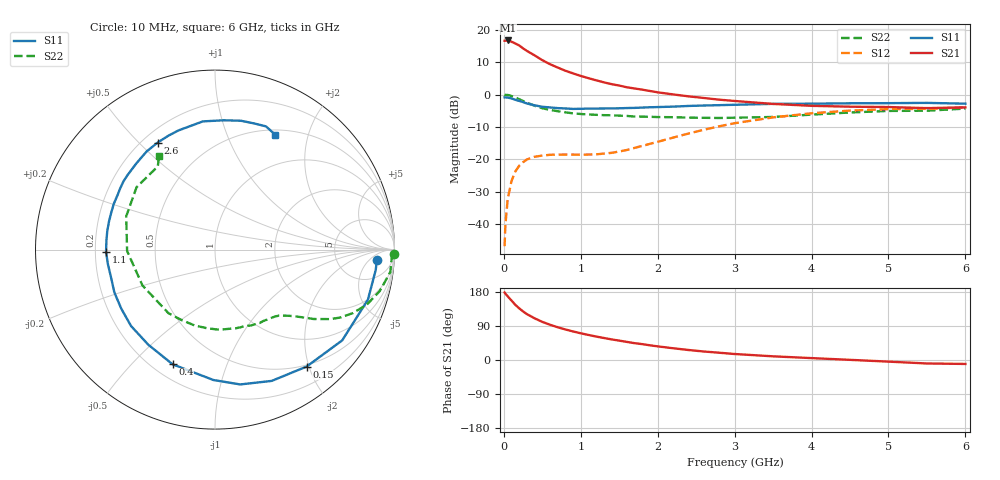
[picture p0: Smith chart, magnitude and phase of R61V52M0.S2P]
! SIEMENS Small Signal Semiconductors
! BFR193
! Si NPN RF Bipolar Junction Transistor in SOT23
! VCE = 1.5 V  IC = 2 mA
! Common Emitter S-Parameters:  May  1996
# GHz  S  MA  R  50
!  f  S11  S21  S12  S22
! GHz  MAG  ANG  MAG  ANG  MAG  ANG  MAG  ANG
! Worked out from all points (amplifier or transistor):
!   36 points, 10 MHz to 6 GHz, reference 50 ohm
!   highest |S21| = 16.7 dB at 50 MHz (marker M1)
!   |S21| within 3 dB of that: start of sweep to 286 MHz
!   unconditionally stable (mu >= 1): 1.143 GHz to 2.093 GHz; 5.877 GHz to end of sweep
!   at 250 MHz: K = 0.23, MSG = 17.5 dB, |S12| = -20.9 dB
!   at 1.4 GHz: K = 1.13, MAG = 8.4 dB, |S12| = -18.0 dB
!   at 6 GHz: K = 1.00, MAG = -0.2 dB, |S12| = -4.0 dB
!   S11 on the Smith chart (normalised r, x): 10 MHz: 14, -9; 150 MHz: 0.47, -1.96; 400 MHz: 0.28, -0.66; 1.1 GHz: 0.24, -0.01; 2.6 GHz: 0.26, +0.57; 6 GHz: 0.56, +1.51
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0.01  0.9037 -3.6  6.736 178.1  0.0046 87.9  0.9989 -1.5
0.02  0.9027 -7.2  6.744 175.1  0.0098 88.1  0.9855 -2.8
0.05  0.8965 -18.1  6.808 168.1  0.0244 80.0  0.9847 -7.3
0.1  0.8707 -35.5  6.506 156.8  0.0466 71.2  0.9467 -14.1
0.15  0.8278 -51.9  6.105 145.4  0.0654 62.4  0.9002 -19.9
0.2  0.797 -66.6  5.694 136.3  0.0798 55.3  0.846 -24.7
0.25  0.7643 -79.4  5.137 128.1  0.0906 49.6  0.7936 -28.5
0.3  0.7266 -90.7  4.702 121.1  0.0998 45.2  0.7497 -31.1
0.4  0.6813 -110.3  4.008 110.0  0.1098 38.5  0.6707 -35.2
0.5  0.6471 -125.1  3.384 100.6  0.1146 34.4  0.6134 -37.9
0.6  0.6324 -137.7  2.932 93.1  0.1177 31.9  0.5795 -39.9
0.7  0.6173 -147.8  2.604 86.4  0.1186 30.7  0.5532 -41.8
0.9  0.5997 -164.7  2.115 75.3  0.1187 31.9  0.512 -45.9
1.1  0.6072 -178.8  1.786 66.1  0.1189 35.8  0.4927 -50.7
1.3  0.6091 170.2  1.541 58.1  0.1229 41.3  0.4807 -55.7
1.6  0.6188 155.7  1.292 47.7  0.1396 51.2  0.4674 -64.9
2.2  0.6505 132.2  1.004 31.0  0.2166 60.2  0.4472 -87.0
2.6  0.6765 118.2  0.884 22.4  0.2863 58.2  0.4374 -105.3
3.5  0.7175 95.4  0.716 9.7  0.444 42.6  0.4508 -153.7
4.5  0.7323 78.6  0.649 0.4  0.5652 22.2  0.5284 159.4
5.5  0.7429 67.5  0.617 -9.2  0.6004 3.7  0.5626 124.5
6  0.7223 62.2  0.634 -10.4  0.6327 -1.4  0.6066 120.9
